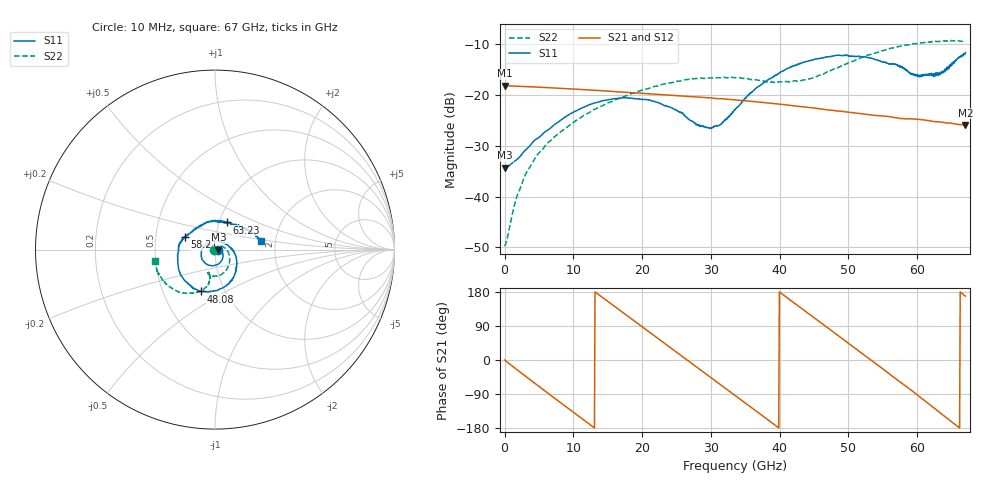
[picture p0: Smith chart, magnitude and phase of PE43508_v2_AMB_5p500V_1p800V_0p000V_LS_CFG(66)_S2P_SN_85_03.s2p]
!Keysight Technologies,N5227A,US51270237,A.10.43.00
!Date: Wednesday, August 22, 2018 17:13:30
!Correction: S11(Full 2 Port(1,3))
!S31(Full 2 Port(1,3))
!S13(Full 2 Port(1,3))
!S33(Full 2 Port(1,3))
!S2P File: Measurements: S11, S31, S13, S33:
# Hz S  dB  R 50
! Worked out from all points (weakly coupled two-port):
!   801 points, 10 MHz to 67 GHz, reference 50 ohm
!   highest |S21| = -18.12 dB at 10 MHz (marker M1); lowest = -25.9 dB at 67 GHz (marker M2)
!   lowest |S11| = -34.3 dB at 93.74 MHz (marker M3), VSWR 1.04, Z = 52 + j0.00888 ohm
!   |S11| at or under -10 dB: start of sweep to end of sweep
!   |S22| runs from -49.8 to -9.2 dB; largest |S21 - S12| = 0.00064
!   S11 on the Smith chart (normalised r, x): 10 MHz: 1.04, -0.00; 48.08 GHz: 0.77, -0.38; 58.21 GHz: 0.71, +0.10; 63.23 GHz: 1.09, +0.34; 67 GHz: 1.69, +0.17
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1e7  -34.22 -1.1  -18.12 -0.2  -18.12 -0.2  -49.79 -177.6
9.37375e7  -34.30 0.3  -18.13 -1.4  -18.14 -1.5  -49.50 169.5
1.852225e9  -32.65 3.5  -18.25 -26.2  -18.25 -26.2  -39.76 85.8
3.02455e9  -30.90 -0.0  -18.32 -42.5  -18.32 -42.5  -35.73 67.8
4.36435e9  -28.92 -7.3  -18.40 -60.9  -18.41 -60.9  -32.60 53.7
7.127688e9  -25.97 -28.7  -18.59 -98.8  -18.59 -98.7  -28.40 32.9
1.123082e10  -22.54 -63.7  -18.90 -154.5  -18.90 -154.4  -24.29 2.9
1.74274e10  -20.53 -114.7  -19.42 122.2  -19.42 122.2  -20.23 -32.5
2.236791e10  -21.51 -156.0  -19.86 55.9  -19.85 56.0  -18.14 -56.5
2.61361e10  -23.87 164.6  -20.19 5.6  -20.18 5.5  -17.02 -73.1
2.973681e10  -26.50 96.8  -20.54 -42.8  -20.54 -42.8  -16.59 -86.4
3.132782e10  -25.88 62.2  -20.71 -64.0  -20.71 -64.0  -16.55 -92.1
3.3505e10  -22.95 22.5  -20.95 -93.5  -20.96 -93.5  -16.56 -98.8
3.836178e10  -16.97 -31.1  -21.57 -158.8  -21.58 -158.7  -17.42 -106.0
4.472582e10  -13.12 -82.7  -22.50 115.4  -22.49 115.4  -16.68 -100.3
4.807532e10  -12.19 -108.3  -23.09 70.1  -23.08 70.0  -14.76 -100.3
5.251341e10  -12.50 -143.5  -23.77 10.0  -23.75 9.9  -12.24 -109.0
5.586291e10  -13.89 -177.4  -24.22 -35.7  -24.20 -36.1  -10.86 -121.5
5.820756e10  -14.77 157.3  -24.65 -67.3  -24.67 -67.6  -10.11 -130.6
6.004979e10  -15.99 124.8  -24.75 -92.8  -24.76 -93.2  -9.85 -138.5
6.323181e10  -15.66 66.6  -25.28 -138.0  -25.33 -138.5  -9.41 -152.7
6.7e10  -11.60 10.0  -25.89 168.5  -25.97 168.5  -9.34 -169.3
